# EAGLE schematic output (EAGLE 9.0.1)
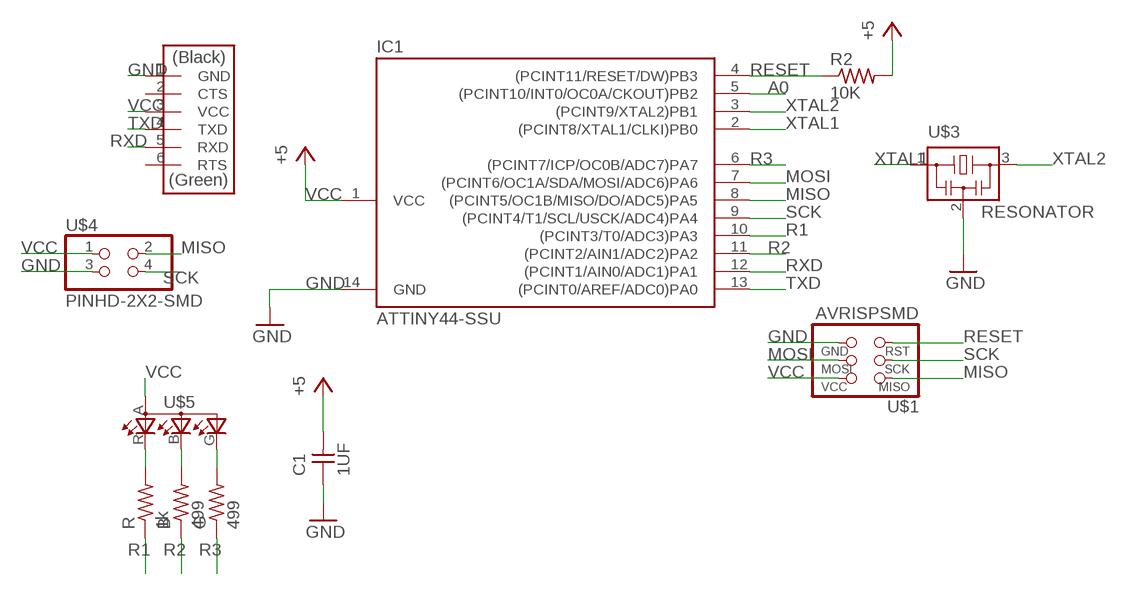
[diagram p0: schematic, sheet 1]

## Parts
B  499  RES-US1206FAB  [R1206FAB]
C1  1UF  CAP-UNPOLARIZEDFAB  [C1206FAB]
G  499  RES-US1206FAB  [R1206FAB]
IC1  ATTINY44-SSU  [SOIC14]
R  1k  RES-US1206FAB  [R1206FAB]
R2  10K  RES-US1206FAB  [R1206FAB]
U$1  AVRISPSMD  [2X03SMD]
U$2  FTDI-SMD-HEADER  [1X06SMD]
U$3  RESONATOR  [EFOBM]
U$4  PINHD-2X2-SMD  [2X02SMD]
U$5  LEDRGBOLD  [P-LCC-4-3]

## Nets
A0: IC1.5((PCINT10/INT0/OC0A/CKOUT)PB2)
GND: C1.1 IC1.14(GND) U$1.6(GND) U$2.1(GND) U$3.2 U$4.3
MISO: IC1.8((PCINT5/OC1B/MISO/DO/ADC5)PA5) U$1.1(MISO) U$4.2
MOSI: IC1.7((PCINT6/OC1A/SDA/MOSI/ADC6)PA6) U$1.4(MOSI)
N$1: R.2 U$5.R(CRED)
N$2: B.2 U$5.B(CBLUE)
N$3: G.2 U$5.G(CGREEN)
R1: IC1.10((PCINT3/T0/ADC3)PA3) R.1
R2: B.1 IC1.11((PCINT2/AIN1/ADC2)PA2)
R3: G.1 IC1.6((PCINT7/ICP/OC0B/ADC7)PA7)
RESET: IC1.4((PCINT11/RESET/DW)PB3) R2.1 U$1.5(RST)
RXD: IC1.12((PCINT1/AIN0/ADC1)PA1) U$2.5(RXD)
SCK: IC1.9((PCINT4/T1/SCL/USCK/ADC4)PA4) U$1.3(SCK) U$4.4
TXD: IC1.13((PCINT0/AREF/ADC0)PA0) U$2.4(TXD)
VCC: C1.2 IC1.1(VCC) R2.2 U$1.2(VCC) U$2.3(VCC) U$4.1 U$5.A(A2) ; supply symbol labelled +5
XTAL1: IC1.2((PCINT8/XTAL1/CLKI)PB0) U$3.1
XTAL2: IC1.3((PCINT9/XTAL2)PB1) U$3.3
Unconnected: U$2.2(CTS) U$2.6(RTS)

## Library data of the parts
B G R R2 = fab:RES-US: Resistor (US Symbol)
C1 = fab:CAP-UNPOLARIZED
IC1 = fab:ATTINY44
U$1 = fab:AVRISP
U$2 = fab:FTDI-SMD-HEADER
U$3 = fab:RESONATOR
U$4 = fab:PINHD-2X2-SMD
U$5 = fab:LEDRGBOLD: OSRAM Hyper Multi TOPLED® Hyper-Bright LED LATB T686 Source: http://www.osram.convergy.de/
